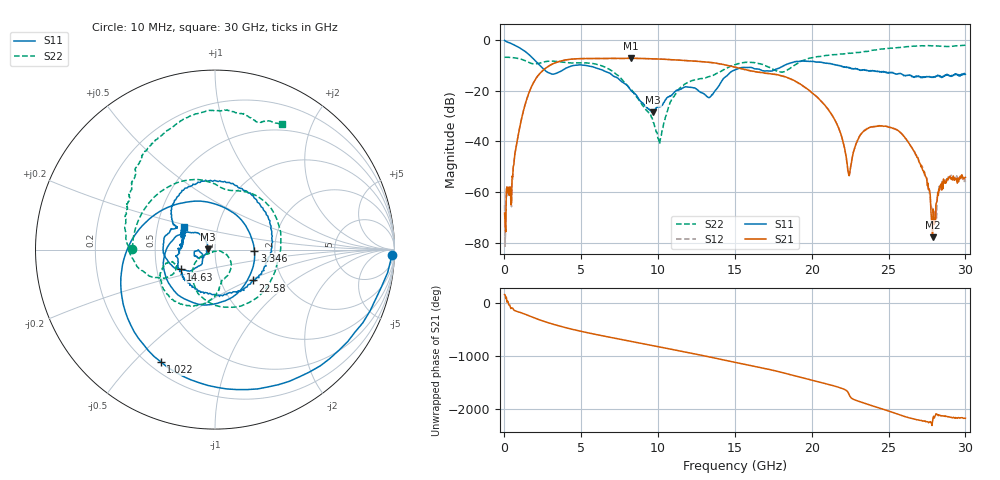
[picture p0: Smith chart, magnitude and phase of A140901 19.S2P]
!  2-Port S-parameters saved by WinCal
! VAR MeasName=S-Parameters (CALIBRATED_DATA) read from VNA (N5244A)
! VAR MeasDate=11/3/2014 9:28:21 AM
! VAR NAME=A140901 19
! VAR FILENAME=A140901 19.S2P
! VAR DATE=11/3/2014 9:28:21 AM
! VAR PHYS_PORTS=1,2
# Hz S RI R 50
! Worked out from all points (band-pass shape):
!   801 points, 10 MHz to 30 GHz, reference 50 ohm
!   highest |S21| = -7.14 dB at 8.22 GHz (marker M1); lowest = -77.7 dB at 27.86 GHz (marker M2)
!   |S21| within 3 dB of the highest: 2.901 GHz to 14.66 GHz (11.75 GHz wide, 134 % of centre)
!   lowest |S11| = -28.5 dB at 9.682 GHz (marker M3), VSWR 1.08, Z = 46.4 + j0.161 ohm
!   |S11| at or under -10 dB: 2.3 GHz to 4.483 GHz (2.183 GHz wide, 64.4 % of centre); 5.291 GHz to 18.2 GHz (12.91 GHz wide, 110 % of centre); 21.76 GHz to end of sweep
!   |S22| runs from -41.0 to -2.0 dB; largest |S21 - S12| = 0.0043
!   S11 on the Smith chart (normalised r, x): 10 MHz: 24, -55; 1.022 GHz: 0.25, -0.60; 3.346 GHz: 1.56, -0.03; 14.63 GHz: 0.66, -0.15; 22.58 GHz: 1.42, -0.53; 30 GHz: 0.69, +0.18
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1e7  0.9863 -0.0303  -0.000379 7.81e-05  -0.00037 -0.000409  -0.4603 0.0046
1.022162e9  -0.3026 -0.6252  -0.0208 -0.00313  -0.0208 -0.00312  -0.2007 0.3765
2.146788e9  -0.2667 0.2338  0.0867 0.1721  0.0866 0.172  0.0993 0.3293
3.346388e9  0.2199 -0.00782  0.2369 -0.2722  0.2375 -0.2727  0.3517 0.1465
5.033325e9  -0.2281 -0.2295  -0.4281 -0.0637  -0.4282 -0.0625  0.2843 -0.2149
6.645288e9  -0.2276 0.0627  -0.012 0.4344  -0.0123 0.4338  -0.0566 -0.2786
8.219762e9  -0.0709 0.0747  0.4391 0.0153  0.4377 0.0152  -0.0912 -0.0563
9.681775e9  -0.0375 0.00174  0.0642 -0.4221  0.0651 -0.4213  -0.0176 -0.0161
1.001916e10  -0.0467 -0.0161  -0.0772 -0.4178  -0.0771 -0.4174  -0.00608 -0.00956
1.125625e10  -0.0919 -0.048  -0.401 -0.0614  -0.4018 -0.061  0.0813 -0.0559
1.271826e10  -0.0955 -0.0051  -0.0901 0.3675  -0.0895 0.3677  0.0492 -0.1664
1.463012e10  -0.1917 -0.1104  0.3041 -0.0717  0.3025 -0.072  -0.045 -0.2917
1.5005e10  -0.2447 -0.0838  0.2378 -0.1721  0.2344 -0.1737  -0.1026 -0.3122
1.721676e10  -0.2131 0.1206  -0.2157 -0.0398  -0.2147 -0.0397  -0.283 -0.082
2.002832e10  0.0797 0.3744  0.0882 -0.0226  0.0884 -0.0217  -0.4438 -0.076
2.257748e10  0.211 -0.1719  0.00371 0.000482  0.00379 0.00047  -0.4853 0.2653
2.336471e10  0.0431 -0.2566  0.0012 -0.0157  0.00118 -0.0159  -0.4636 0.3685
2.501416e10  -0.1924 -0.1134  -0.00958 0.0165  -0.0098 0.017  -0.3421 0.6008
2.681356e10  -0.1868 0.0249  0.00385 -0.00366  0.00403 -0.00366  -0.0757 0.7628
2.786321e10  -0.1756 0.0637  3.6e-05 -0.000124  -5.25e-05 -0.000318  0.1263 0.7618
2.85005e10  -0.1742 0.0821  0.00135 0.000811  0.00132 0.000978  0.2179 0.7217
3e10  -0.17 0.1259  0.00189 -0.000546  0.00153 -0.000424  0.3756 0.6995
